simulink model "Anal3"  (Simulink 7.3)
settings: Solver=ode45  StartTime=0.0  StopTime=10.0  RelTol=1e-3
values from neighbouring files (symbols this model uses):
  Kp = om^2    (= 1.44)    [run.m]
  Kp3 = [0.3042  3.4539  0.5105  0.0711 -0.2670]    [run.m]
  Kr = 2*zt*om    (= 0.336)    [run.m]
undefined symbols (not defined in the file or in its folder): An, Bn, Cn, Dn

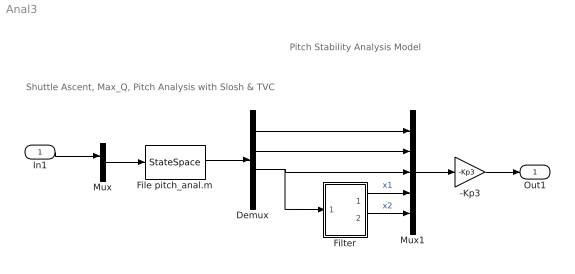
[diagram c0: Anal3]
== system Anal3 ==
  note: Shuttle Ascent, Max_Q, Pitch Analysis with Slosh & TVC
  note: Pitch Stability Analysis Model
  In1 : Inport  OutDataType=sfix(16)  OutScaling=2^0
  -Kp3 : Gain  Gain=-Kp3  Multiplication=Matrix(K*u)  ParameterDataType=sfix(16)  ParameterScaling=2^0  OutDataType=sfix(16)  OutScaling=2^0
  Demux : Demux
  File pitch_anal.m : StateSpace  A=An  B=Bn  C=Cn  D=Dn
  Filter : Subsystem
  Mux : Mux  Inputs=2
  Mux1 : Mux  Inputs=5
  Out1 : Outport  OutDataType=sfix(16)  OutScaling=2^0
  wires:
  Mux/1 -> File pitch_anal.m/1
  File pitch_anal.m/1 -> Demux/1
  Demux/1 -> Mux1/1
  Demux/2 -> Mux1/2
  Mux1/1 -> -Kp3/1
  In1/1 -> Mux/1
  -Kp3/1 -> Out1/1
  Filter/1(ai) -> Mux1/4  "x1"
  Filter/2(aii) -> Mux1/5  "x2"
  Demux/3 -> Mux1/3, Filter/1(a)

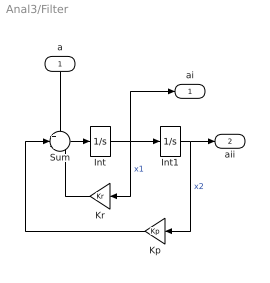
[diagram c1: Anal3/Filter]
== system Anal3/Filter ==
  a : Inport  OutDataType=sfix(16)  OutScaling=2^0
  Int : Integrator
  Int1 : Integrator
  Kp : Gain  Gain=Kp  ParameterDataType=sfix(16)  ParameterScaling=2^0  OutDataType=sfix(16)  OutScaling=2^0
  Kr : Gain  Gain=Kr  ParameterDataType=sfix(16)  ParameterScaling=2^0  OutDataType=sfix(16)  OutScaling=2^0
  Sum : Sum  Inputs=+--  OutDataType=sfix(16)  OutScaling=2^0
  ai : Outport  OutDataType=sfix(16)  OutScaling=2^0
  aii : Outport  Port=2  OutDataType=sfix(16)  OutScaling=2^0
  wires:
  Int/1 -> Int1/1, Kr/1, ai/1  "x1"
  Sum/1 -> Int/1
  Int1/1 -> Kp/1, aii/1  "x2"
  Kr/1 -> Sum/3
  Kp/1 -> Sum/2
  a/1 -> Sum/1
